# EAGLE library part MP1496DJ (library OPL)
High-Efficiency,2A，16V,500kHz Synchronous,Step-Down Converter http://html.alldatasheetcn.com/html-pdf/551584/MPS/MP1496DJ/55/1/MP1496DJ.html
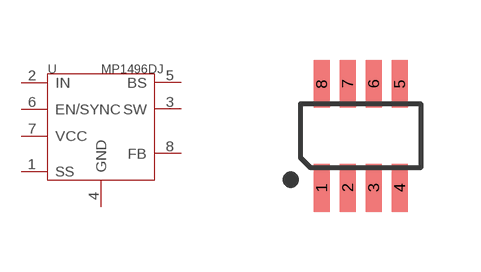
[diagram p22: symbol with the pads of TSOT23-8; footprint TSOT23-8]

Designator prefix U

## MP1496DJ-310030121  [TSOT23-8]
1  SS
2  IN
3  SW
4  GND
5  BS
6  EN/SYNC
7  VCC
8  FB

## Footprint TSOT23-8 (pad centres in mm)
smd 0.4 x 1.2: 1 -0.975,-1.3; 2 -0.325,-1.3; 3 0.325,-1.3; 4 0.975,-1.3; 5 0.975,1.3; 6 0.325,1.3; 7 -0.325,1.3; 8 -0.975,1.3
